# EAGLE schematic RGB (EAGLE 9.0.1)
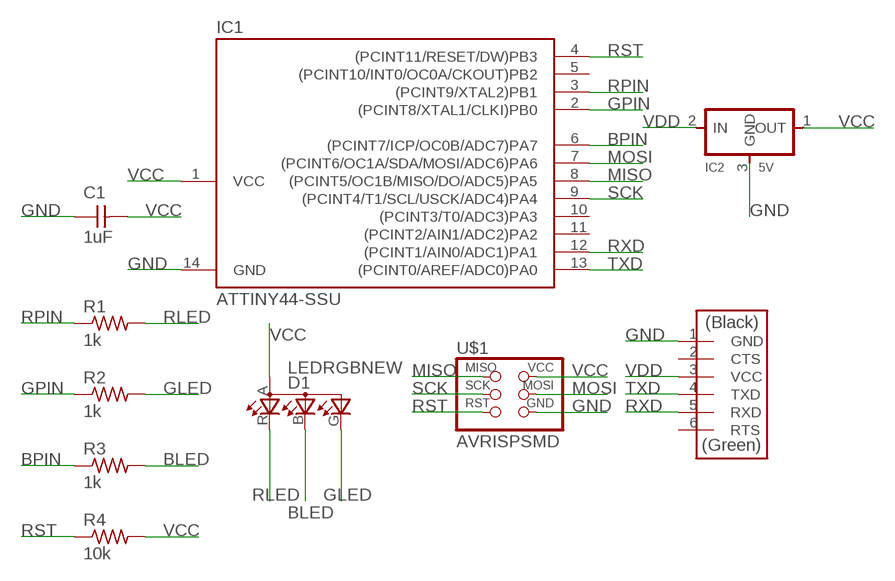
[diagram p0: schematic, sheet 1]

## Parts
C1  1uF  CAP-UNPOLARIZEDFAB  [C1206FAB]
D1  LEDRGBNEW  [P-LCC-4]
IC1  ATTINY44-SSU  [SOIC14]
IC2  5V  REGULATORSOT23  [SOT23]
R1  1k  RES-US1206FAB  [R1206FAB]
R2  1k  RES-US1206FAB  [R1206FAB]
R3  1k  RES-US1206FAB  [R1206FAB]
R4  10k  RES-US1206FAB  [R1206FAB]
U$1  AVRISPSMD  [2X03SMD]
U$2  FTDI-SMD-HEADER  [1X06SMD]

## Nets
BLED: D1.B(CBLUE) R3.2
BPIN: IC1.6((PCINT7/ICP/OC0B/ADC7)PA7) R3.1
GLED: D1.G(CGREEN) R2.2
GND: C1.1 IC1.14(GND) IC2.3(GND) U$1.6(GND) U$2.1(GND)
GPIN: IC1.2((PCINT8/XTAL1/CLKI)PB0) R2.1
MISO: IC1.8((PCINT5/OC1B/MISO/DO/ADC5)PA5) U$1.1(MISO)
MOSI: IC1.7((PCINT6/OC1A/SDA/MOSI/ADC6)PA6) U$1.4(MOSI)
RLED: D1.R(CRED) R1.2
RPIN: IC1.3((PCINT9/XTAL2)PB1) R1.1
RST: IC1.4((PCINT11/RESET/DW)PB3) R4.1 U$1.5(RST)
RXD: IC1.12((PCINT1/AIN0/ADC1)PA1) U$2.5(RXD)
SCK: IC1.9((PCINT4/T1/SCL/USCK/ADC4)PA4) U$1.3(SCK)
TXD: IC1.13((PCINT0/AREF/ADC0)PA0) U$2.4(TXD)
VCC: C1.2 D1.A(A2) IC1.1(VCC) IC2.1(OUT) R4.2 U$1.2(VCC)
VDD: IC2.2(IN) U$2.3(VCC)
Unconnected: IC1.5((PCINT10/INT0/OC0A/CKOUT)PB2) IC1.10((PCINT3/T0/ADC3)PA3) IC1.11((PCINT2/AIN1/ADC2)PA2) U$2.2(CTS) U$2.6(RTS)

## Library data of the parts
C1 = fab:CAP-UNPOLARIZED
D1 = fab:LEDRGBNEW
IC1 = fab:ATTINY44
IC2 = fab:REGULATOR
R1-R4 = fab:RES-US: Resistor (US Symbol)
U$1 = fab:AVRISP
U$2 = fab:FTDI-SMD-HEADER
